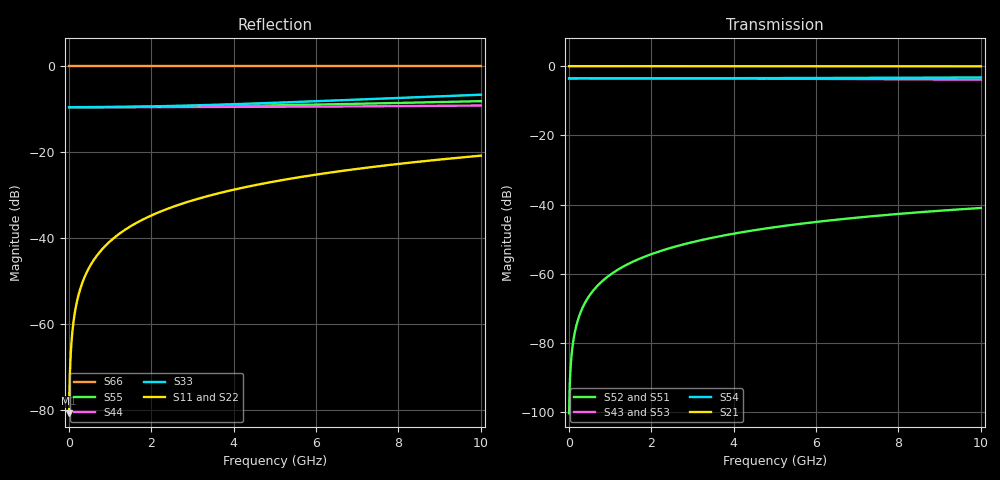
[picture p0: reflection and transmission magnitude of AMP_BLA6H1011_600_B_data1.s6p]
! Created Mon Apr 26 22:19:58 2010
# ghz S ma R 50
! 6 Port Network Data from SP1.SP block
! freq  magS11  angS11  magS12  angS12  magS13  angS13  magS14  angS14
!  magS15  angS15  magS16  angS16
!  magS21  angS21  magS22  angS22
!  magS23  angS23  magS24  angS24  magS25  angS25  magS26  angS26
!  magS31  angS31  magS32  angS32  magS33  angS33  magS34  angS34
!  magS35  angS35  magS36  angS36
!  magS41  angS41  magS42  angS42
!  magS43  angS43  magS44  angS44  magS45  angS45  magS46  angS46
!  magS51  angS51  magS52  angS52  magS53  angS53  magS54  angS54
!  magS55  angS55  magS56  angS56
!  magS61  angS61  magS62  angS62
!  magS63  angS63  magS64  angS64  magS65  angS65  magS66  angS66
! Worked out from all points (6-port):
!   1000 points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, 10 MHz to 10 GHz, reference 50 ohm
!   strongest paths, dB at 10 MHz, 2.51 GHz, 5.01 GHz, 7.51 GHz, 10 GHz:
!     S21: 0.0, 0.0, 0.0, 0.0, 0.0
!     S54: -3.5, -3.5, -3.4, -3.4, -3.3
!     S43: -3.5, -3.5, -3.6, -3.7, -3.9
!     S53: -3.5, -3.6, -3.7, -4.0, -4.3
!     S52: -100.4, -52.4, -46.5, -43.2, -41.0
!     S51: -100.4, -52.4, -46.5, -43.2, -41.0
!   lowest |S11| = -80.8 dB at 10 MHz (marker M1), VSWR 1.00, Z = 50 + j0.00913 ohm
!   |S11| at or under -10 dB: start of sweep to end of sweep
